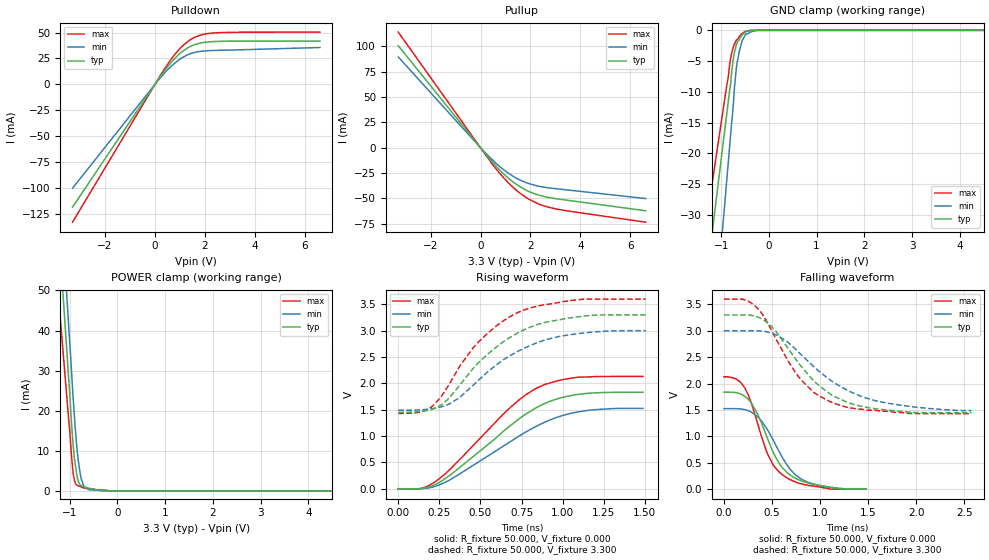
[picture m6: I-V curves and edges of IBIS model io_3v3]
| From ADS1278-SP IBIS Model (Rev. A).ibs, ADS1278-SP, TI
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[Model]   io_3v3
Model_type I/O
Vinl=0.990E+00
Vinh=2.310E+00
Vref=0.000E+00
Rref=1.000E+06
Cref=2.000E-11
Vmeas=1.650E+00
C_comp   698.00E-15   698.00E-15   698.00E-15
[Voltage Range]   3.300E+00   3.000E+00   3.600E+00
[POWER Clamp Reference]   3.300E+00   3.000E+00   3.600E+00
[GND Clamp Reference]   0.000E+00   0.000E+00   0.000E+00
[Pullup Reference]   3.300E+00   3.000E+00   3.600E+00
[Pulldown Reference]   0.000E+00   0.000E+00   0.000E+00
[Temperature Range]   25   105   -40
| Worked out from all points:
|   slope of the pulldown table from 0 to 0.495 V, typ, clamps not added: 29.7 ohm
|   slope of the pullup table from 0 to 0.495 V, typ, clamps not added: 33.5 ohm
|   GND clamp passes 1 mA (typ) near -0.58 V on its own axis
|   POWER clamp passes 1 mA (typ) near -0.69 V on its own axis
|   rising waveform, R_fixture 50.000, V_fixture 0.000: 20-80 % time 441ps typ, 477ps min, 410ps max; typ from 0 V to 1.83 V
|   falling waveform, R_fixture 50.000, V_fixture 0.000: 20-80 % time 288ps typ, 307ps min, 255ps max; typ from 1.84 V to 0.009 V
|   rising waveform, R_fixture 50.000, V_fixture 3.300: 20-80 % time 376ps typ, 393ps min, 344ps max; typ from 1.45 V to 3.3 V
|   falling waveform, R_fixture 50.000, V_fixture 3.300: 20-80 % time 527ps typ, 666ps min, 466ps max; typ from 3.3 V to 1.45 V
[GND Clamp]
-3.3V     -166.8mA   -245mA     -135mA
-880mV    -13.44mA   -24.22mA   -8.856mA
-800mV    -8.665mA   -16.95mA   -4.521mA
-780mV    -6.944mA   -15.06mA   -3.774mA
-740mV    -4.453mA   -11.58mA   -2.619mA
-720mV    -3.573mA   -9.253mA   -2.215mA
-680mV    -2.332mA   -6.037mA   -1.577mA
-620mV    -1.51mA    -3.442mA   -1.003mA
-560mV    -728.8uA   -1.695mA   -489.3uA
-480mV    -226.7uA   -576.2uA   -145.5uA
-240mV    -8.516uA   0A         0A
6.6V      0A         0A         0A
[Power Clamp]
-3.3V     434.1mA    475.4mA    345.4mA
-1.02V    27.74mA    40.96mA    17.58mA
-1V       24.62mA    37.15mA    15.18mA
-940mV    13.28mA    25.48mA    5.706mA
-920mV    10.34mA    21.77mA    3.767mA
-880mV    6.422mA    15.02mA    1.901mA
-820mV    2.374mA    7.577mA    1.236mA
-760mV    1.345mA    3.107mA    1.011mA
-720mV    1.136mA    1.713mA    794.6uA
-560mV    559.2uA    228.2uA    565uA
-160mV    0A         0A         0A
6.62V     0A         0A         0A
[Pullup]
-3.3V     100.7mA    89.62mA    114.1mA
300mV     -9.079mA   -7.591mA   -10.12mA
500mV     -15.02mA   -12.39mA   -17.15mA
920mV     -25.57mA   -21.58mA   -29.49mA
1.24V     -32.51mA   -27.06mA   -37.51mA
1.58V     -38.36mA   -31.77mA   -44.79mA
1.9V      -42.7mA    -35.06mA   -50.19mA
2.3V      -46.47mA   -37.76mA   -55.14mA
2.84V     -49.58mA   -39.9mA    -59.38mA
6.62V     -62.16mA   -50.11mA   -73.44mA
[Pulldown]
-3.3V     -118.7mA   -100.5mA   -133.3mA
200mV     7.178mA    6.01mA     8.189mA
540mV     18.04mA    15.14mA    20.68mA
800mV     25.17mA    20.71mA    29.12mA
1.08V     31.46mA    25.61mA    36.67mA
1.32V     35.41mA    28.7mA     41.6mA
1.5V      37.59mA    30.27mA    44.4mA
1.78V     39.72mA    31.75mA    47.3mA
2.36V     41.37mA    32.77mA    49.71mA
6.6V      41.75mA    35.64mA    50.53mA
[Rising Waveform]
R_fixture = 50.000
V_fixture = 0.000
V_fixture_min = 0.000
V_fixture_max = 0.000
|  time   V(typ)   V(min)   V(max)
0s        0V         0V         0V
142.5ps   4.406mV    899uV      10.79mV
235ps     95.83mV    56.33mV    156.2mV
352.5ps   349.1mV    238.8mV    487.7mV
672.5ps   1.175V     875.6mV    1.517V
772.5ps   1.41V      1.071V     1.775V
850ps     1.556V     1.201V     1.923V
962.5ps   1.701V     1.352V     2.043V
1.087ns   1.788V     1.455V     2.115V
1.488ns   1.831V     1.525V     2.131V
[Falling Waveform]
R_fixture = 50.000
V_fixture = 0.000
V_fixture_min = 0.000
V_fixture_max = 0.000
|  time   V(typ)   V(min)   V(max)
0s        1.837V     1.525V     2.131V
170ps     1.806V     1.521V     2.029V
280ps     1.645V     1.465V     1.658V
362.5ps   1.373V     1.349V     1.169V
455ps     950.2mV    1.12V      663.2mV
525ps     650.8mV    885.3mV    428.3mV
612.5ps   396.3mV    585.8mV    266.2mV
735ps     215.9mV    287.7mV    144.9mV
875ps     116.8mV    131.5mV    74.41mV
1.48ns    8.749mV    0V         0V
[Rising Waveform]
R_fixture = 50.000
V_fixture = 3.300
V_fixture_min = 3.000
V_fixture_max = 3.600
|  time   V(typ)   V(min)   V(max)
0s        1.45V      1.489V     1.43V
135ps     1.468V     1.497V     1.456V
207.5ps   1.509V     1.521V     1.567V
310ps     1.724V     1.607V     1.983V
472.5ps   2.342V     2.014V     2.734V
597.5ps   2.691V     2.353V     3.092V
725ps     2.955V     2.604V     3.341V
852.5ps   3.123V     2.78V      3.471V
1.007ns   3.223V     2.905V     3.554V
1.505ns   3.3V       3V         3.6V
[Falling Waveform]
R_fixture = 50.000
V_fixture = 3.300
V_fixture_min = 3.000
V_fixture_max = 3.600
|  time   V(typ)   V(min)   V(max)
0s        3.3V       3V         3.6V
262.5ps   3.299V     3V         3.551V
435ps     3.178V     2.985V     3.211V
557.5ps   2.95V      2.911V     2.791V
795ps     2.346V     2.561V     2.086V
932.5ps   2.057V     2.325V     1.836V
1.095ns   1.817V     2.082V     1.665V
1.328ns   1.619V     1.835V     1.536V
1.585ns   1.522V     1.672V     1.491V
2.575ns   1.45V      1.489V     1.43V
[Ramp]
dV/dt_r   1.097E+00/4.402E-10   9.158E-01/4.763E-10   1.279E+00/4.094E-10
dV/dt_f   1.110E+00/5.265E-10   9.065E-01/6.644E-10   1.302E+00/4.649E-10
R_load = 50
